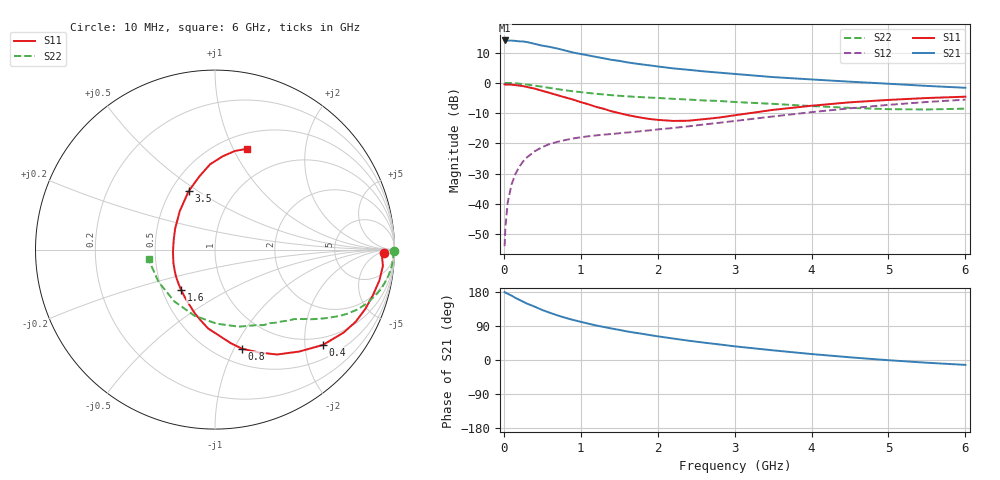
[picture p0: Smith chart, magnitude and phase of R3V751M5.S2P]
! SIEMENS Small Signal Semiconductors
! BFR181
! Si NPN RF Bipolar Junction Transistor in SOT23
! VCE = 0.75 V  IC = 1.5 mA
! Common Emitter S-Parameters:  May  1996
# GHz  S  MA  R  50
!  f  S11  S21  S12  S22
! GHz  MAG  ANG  MAG  ANG  MAG  ANG  MAG  ANG
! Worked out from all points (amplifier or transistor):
!   36 points, 10 MHz to 6 GHz, reference 50 ohm
!   highest |S21| = 14.0 dB at 10 MHz (marker M1)
!   |S21| within 3 dB of that: start of sweep to 747.2 MHz
!   unconditionally stable (mu >= 1): 1.622 GHz to 3.88 GHz
!   at 250 MHz: K = 0.21, MSG = 19.8 dB, |S12| = -26.0 dB
!   at 1.4 GHz: K = 0.92, MSG = 12.3 dB, |S12| = -16.9 dB
!   at 6 GHz: K = 0.92, MSG = 2.0 dB, |S12| = -5.6 dB
!   S11 on the Smith chart (normalised r, x): 10 MHz: 29, -10; 400 MHz: 0.81, -2.41; 800 MHz: 0.66, -1.08; 1.6 GHz: 0.62, -0.31; 3.5 GHz: 0.61, +0.46; 6 GHz: 0.66, +1.13
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0.01  0.9409 -1.2  5.006 179.2  0.002 97.1  0.9964 -0.5
0.02  0.9306 -1.9  4.994 177.8  0.0041 84.4  0.9925 -1.1
0.05  0.9399 -5.6  4.98 174.9  0.0105 88.0  0.9941 -2.8
0.1  0.9319 -10.7  4.977 170.0  0.0209 84.0  0.9893 -5.3
0.15  0.9152 -16.3  4.921 163.9  0.0311 79.1  0.9789 -8.2
0.25  0.881 -27.1  4.816 154.0  0.0502 72.7  0.9533 -13.0
0.3  0.8529 -32.8  4.716 148.9  0.0585 70.7  0.935 -15.3
0.4  0.8021 -41.5  4.402 140.9  0.0738 65.2  0.8987 -19.4
0.5  0.737 -50.4  4.109 131.9  0.0866 60.7  0.861 -22.8
0.6  0.679 -59.4  3.91 124.5  0.0978 56.9  0.8216 -25.7
0.7  0.6231 -66.9  3.671 117.6  0.1061 53.9  0.7845 -28.2
0.8  0.5731 -74.6  3.407 111.3  0.1134 51.3  0.7511 -30.1
0.9  0.5284 -80.5  3.164 105.8  0.1204 49.5  0.7253 -31.8
1.1  0.4417 -94.9  2.834 95.9  0.1308 46.8  0.6793 -34.7
1.3  0.3715 -107.8  2.535 87.1  0.1393 45.6  0.6404 -37.1
1.6  0.2942 -129.8  2.181 75.4  0.1507 45.4  0.5988 -40.3
2.2  0.2345 -177.1  1.731 56.7  0.1794 47.1  0.5433 -47.6
2.8  0.2665 141.8  1.471 41.1  0.2185 48.1  0.501 -57.1
3.5  0.3571 114.3  1.242 25.5  0.2779 46.6  0.4487 -73.1
4.5  0.476 93.3  1.043 7.1  0.379 39.1  0.3852 -107.6
5.5  0.5604 78.6  0.888 -7.2  0.4822 26.8  0.3624 -150.2
6  0.5896 72.4  0.827 -12.9  0.527 19.6  0.3742 -171.6
